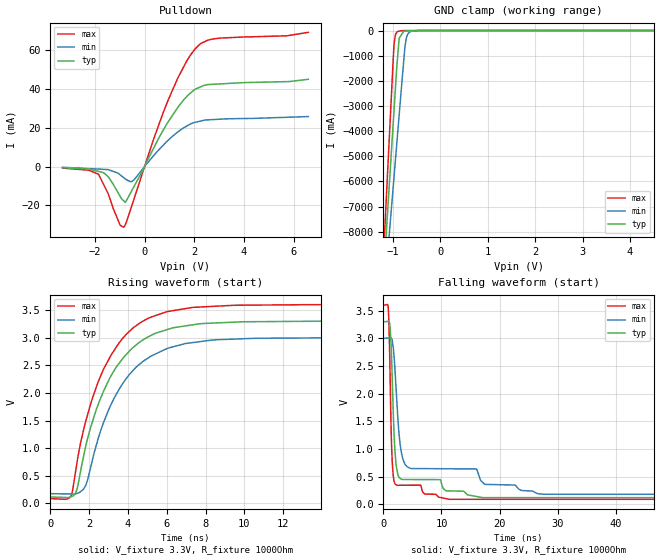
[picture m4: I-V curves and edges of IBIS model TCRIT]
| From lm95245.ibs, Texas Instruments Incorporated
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|   Model T_CRITB
[Model]   TCRIT
Model_type   Open_drain
Polarity   Non-Inverting
Enable   Active-Low
Vmeas = 1.65
Vref = 1.65
Cref = 15pF
Rref = 1000
|   typ   min   max
|   (nom PVT)   (fast PVT)   (slow PVT)
| Where   nom PVT is  Nominal Process, 3.3V, 27C
|   Fast PVT is Strong Process, 3.6V, -40C
|   Slow PVT is Weak Process, 3.0V, 125C
C_comp   0.8853p   0.8722p   0.9155p
|C_comp (ON state)   0.8853p   0.8722p   0.9155p
|C_comp (OFF state)   0.9114p   0.8957p   0.9208p
[Voltage Range]   3.3   3   3.6
[Temperature Range]   27   125   -40
[Pullup Reference]   3.3   3   3.6
[Pulldown Reference]   0   0   0
[Power Clamp Reference]   3.3   3   3.6
[GND Clamp Reference]   0   0   0
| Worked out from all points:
|   slope of the pulldown table from 0 to 0.495 V, typ, clamps not added: 38.7 ohm
|   GND clamp passes 1 mA (typ) near -0.45 V on its own axis
|   falling waveform, V_fixture 3.3V, R_fixture 1000Ohm: 20-80 % time 751ps typ, 1.65ns min, 471ps max; typ from 3.3 V to 0.117 V
|   rising waveform, V_fixture 3.3V, R_fixture 1000Ohm: 20-80 % time 2.17ns typ, 2.2ns min, 2.13ns max; typ from 0.117 V to 3.3 V
[Pulldown]
|   Voltage   I(typ)   I(min)   I(max)
-3.3V     -602.7uA   -366.2uA   -793.4uA
-1.853V   -2.5mA     -1.306mA   -3.943mA
-1.461V   -5.236mA   -1.577mA   -14.09mA
-986.8mV  -15.24mA   -4.237mA   -30.11mA
-845.6mV  -17.59mA   -5.675mA   -31.26mA
-768.1mV  -18.44mA   -6.464mA   -29.77mA
-434.7mV  -10.53mA   -7.009mA   -17.09mA
942.1mV   22.95mA    13.48mA    34.07mA
1.684V    35.93mA    20.79mA    54.15mA
2.031V    39.81mA    22.79mA    60.65mA
2.744V    42.42mA    24.23mA    65.78mA
6.59V     45mA       25.78mA    69.23mA
[GND Clamp]
|   Voltage   I(typ)   I(min)   I(max)
-3.3V     -72.96A    -59.34A    -89.27A
-1.259V   -11.62A    -12.3A     -11.25A
-1.065V   -5.822A    -7.852A    -3.87A
-974.5mV  -3.129A    -5.788A    -530.5mA
-949.7mV  -2.396A    -5.224A    -196.1mA
-900.2mV  -1.047A    -4.096A    -43.84mA
-867.1mV  -303.1mA   -3.343A    -23.24mA
-747.5mV  -22.66mA   -684.7mA   -2.292mA
-722.7mV  -20.86mA   -356.9mA   -1.692mA
-685.6mV  -18.16mA   -142.6mA   -1.082mA
-599mV    -11.86mA   -24.26mA   -694uA
6.59V     0A         0A         0A
[Ramp]
R_load = 1000
|   typ   min   max
dV/dt_r   1.90955/2.17373e-09   1.69361/2.19644e-09   2.10728/2.12902e-09
dV/dt_f   1.90955/7.50937e-10   1.69361/1.63827e-09   2.10728/4.70974e-10
[Falling Waveform]
V_fixture = 3.3V
V_fixture_min = 3V
V_fixture_max = 3.6V
R_fixture = 1000Ohm
C_fixture = 0F
|   Time   V(typ)   V(min)   V(max)
0s        3.3V       3V         3.6V
823ps     3.307V     3.007V     3.569V
1.13ns    3.235V     3.009V     2.441V
1.551ns   2.17V      2.936V     714.7mV
1.907ns   1.109V     2.569V     393mV
2.257ns   664.2mV    1.962V     344.4mV
3.005ns   459.4mV    991.9mV    342.6mV
4.066ns   446.5mV    678.8mV    342.9mV
26.49ns   118.3mV    191.8mV    88.41mV
100ns     117.4mV    177.3mV    87.86mV
[Rising Waveform]
V_fixture = 3.3V
V_fixture_min = 3V
V_fixture_max = 3.6V
R_fixture = 1000Ohm
C_fixture = 0F
|   Time   V(typ)   V(min)   V(max)
0s        117.4mV    177.3mV    87.86mV
1.07ns    120.8mV    172.1mV    137.5mV
1.385ns   269.3mV    182.6mV    758.8mV
1.712ns   849.3mV    257.4mV    1.324V
1.938ns   1.196V     445.9mV    1.626V
2.506ns   1.828V     1.22V      2.231V
3.545ns   2.535V     2.064V     2.906V
5.181ns   3.039V     2.665V     3.37V
7.322ns   3.232V     2.91V      3.546V
100ns     3.3V       3V         3.6V
